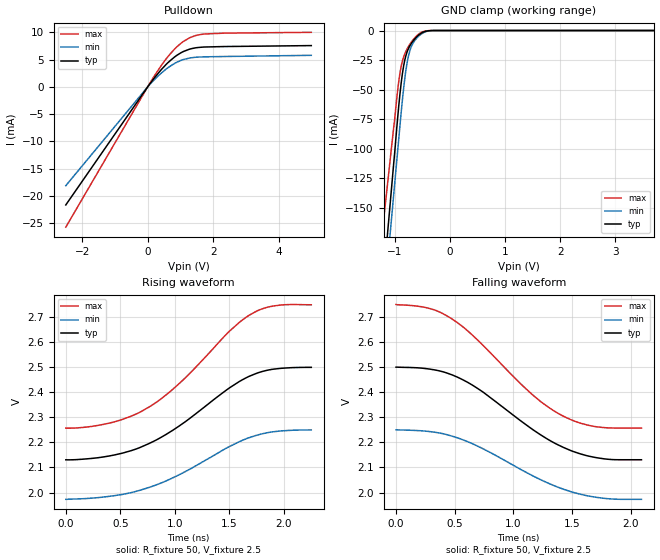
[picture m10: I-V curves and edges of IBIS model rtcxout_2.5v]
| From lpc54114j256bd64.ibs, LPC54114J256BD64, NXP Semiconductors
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[Model]   rtcxout_2.5v
Model_type Open_drain
Vref=2.500E+00
Rref=1.000E+03
Cref=0.000E+00
Vmeas=1.250E+00
C_comp   1.410E-12   1.370E-12   1.450E-12
[Voltage Range]   2.500E+00   2.250E+00   2.750E+00
[POWER Clamp Reference]   2.500E+00   2.250E+00   2.750E+00
[GND Clamp Reference]   0.000E+00   0.000E+00   0.000E+00
[Pullup Reference]   2.500E+00   2.250E+00   2.750E+00
[Pulldown Reference]   0.000E+00   0.000E+00   0.000E+00
[Temperature Range]   25   85   -40
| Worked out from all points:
|   slope of the pulldown table from 0 to 0.375 V, typ, clamps not added: 131 ohm
|   GND clamp passes 1 mA (typ) near -0.46 V on its own axis
|   rising waveform, R_fixture 50, V_fixture 2.5: 20-80 % time 724ps typ, 736ps min, 704ps max; typ from 2.13 V to 2.5 V
|   falling waveform, R_fixture 50, V_fixture 2.5: 20-80 % time 663ps typ, 691ps min, 658ps max; typ from 2.5 V to 2.13 V
[GND Clamp]
-2.5V     -900.5mA   -901.8mA   -716.7mA
-1.02V    -113.3mA   -139.7mA   -82.6mA
-940mV    -70.45mA   -98.58mA   -47.83mA
-920mV    -60.54mA   -88.17mA   -40.61mA
-880mV    -43.29mA   -67.93mA   -29.64mA
-840mV    -30.35mA   -49.57mA   -22.62mA
-780mV    -18.7mA    -28.5mA    -16mA
-740mV    -14.25mA   -19.5mA    -12.71mA
-680mV    -9.646mA   -11.73mA   -8.599mA
-520mV    -2.254mA   -3.006mA   -1.608mA
-300mV    0A         0A         0A
5V        0A         0A         0A
[Pulldown]
-2.5V     -21.66mA   -18.12mA   -25.74mA
0V        0A         0A         0A
180mV     1.454mA    1.174mA    1.781mA
600mV     4.34mA     3.437mA    5.421mA
820mV     5.479mA    4.296mA    6.92mA
1.02V     6.278mA    4.874mA    8.024mA
1.32V     6.998mA    5.342mA    9.113mA
1.72V     7.322mA    5.519mA    9.71mA
5V        7.587mA    5.8mA      10.02mA
[Rising Waveform]
R_fixture = 50
V_fixture = 2.5
V_fixture_min = 2.25
V_fixture_max = 2.75
0s        2.131V     1.973V     2.257V
380ps     2.145V     1.984V     2.275V
670ps     2.178V     2.008V     2.319V
830ps     2.21V      2.031V     2.36V
990ps     2.251V     2.061V     2.416V
1.14ns    2.297V     2.094V     2.477V
1.5ns     2.418V     2.184V     2.645V
1.68ns    2.464V     2.219V     2.708V
1.9ns     2.493V     2.243V     2.745V
2.25ns    2.5V       2.25V      2.75V
[Falling Waveform]
R_fixture = 50
V_fixture = 2.5
V_fixture_min = 2.25
V_fixture_max = 2.75
0s        2.5V       2.25V      2.75V
280ps     2.493V     2.243V     2.735V
480ps     2.469V     2.224V     2.691V
730ps     2.404V     2.177V     2.592V
1.17ns    2.249V     2.065V     2.387V
1.29ns    2.213V     2.038V     2.343V
1.43ns    2.179V     2.012V     2.303V
1.56ns    2.156V     1.994V     2.278V
1.7ns     2.139V     1.981V     2.263V
2.09ns    2.131V     1.973V     2.257V
[Ramp]
dV/dt_r   2.2159E-01/7.2230E-10   1.6633E-01/7.3410E-10   2.9569E-01/7.0260E-10
dV/dt_f   2.2159E-01/6.6203E-10   1.6633E-01/6.9023E-10   2.9569E-01/6.5750E-10
R_load = 50
